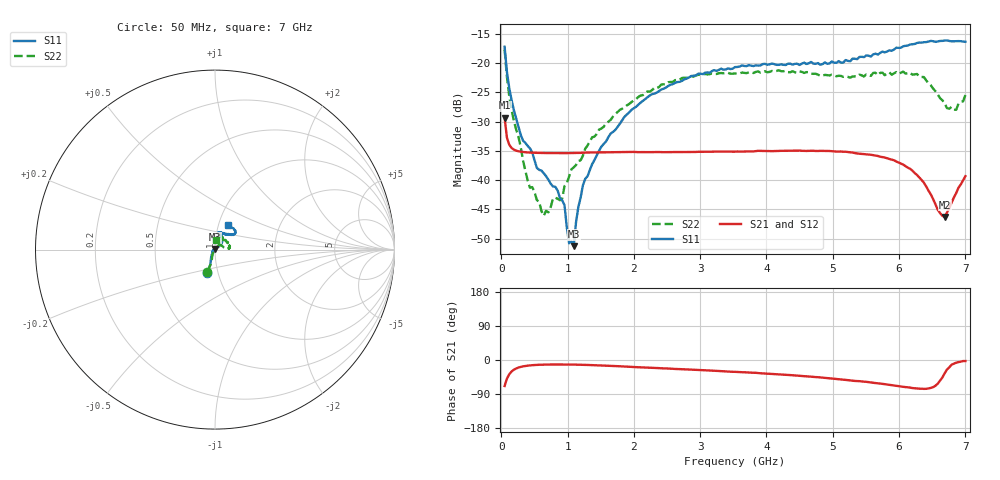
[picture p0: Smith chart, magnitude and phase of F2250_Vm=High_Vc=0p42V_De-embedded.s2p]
! Integrated Device Technology
! Corporate Headquarters
! 6024 Silver Creek Valley Road
! San Jose, CA 95138  USA
! Phone:  1-408-284-8200
! Toll Free:  1-800-223-1366
! Webpage:  http://www.idt.com/
! Timing and RF Division
! 515 Groton Road, Suite 102
! Westford, MA 01886-6024
! Device:  F2250
! Description: Voltage Variable RF Attenuator
! Frequency:  50.0 -  6000.00 MHz
! Package:  3x3 mm Thin QFN Plastic Package: 16 pin
! Ports:  2 RF, 3 DC
!  Pin  1  = GND
!  Pin  2  = NC
!  Pin  3  = RF1  = Port 1
!  Pin  4  = NC
!  Pin  5  = GND
!  Pin  6  = GND
!  Pin  7  = GND
!  Pin  8  = GND
!  Pin  9  = NC
!  Pin 10  = RF2  = Port 2
!  Pin 11  = NC
!  Pin 12  = GND
!  Pin 13  = GND
!  Pin 14  = VCNTRL
!  Pin 15  = VDD
!  Pin 16  = VMODE
! Vcntrl:  0.420 Volts
! Vmode:  +3.300 Volts
! Vdd:  +3.30  Volts
! Current:  1.265 mA
! Data:  The device was measured on a the F2250 evaluation board which has
!  individual transmission lines to the RF pins.  Data was collected
!  using a calibrated network analyzer.  The evaluation board was
!  de-embedded using a TRL calibration technique.
!  The reference plane is the edge of the package pin.
! Misc:  SN 10
!  Action Tracker AT0258
! Date Measured:  2014-11-26
! Date:  2015-10-15  MJV
! Note:
!  Integrated Device Technology supplies this data as a sample of measured
!  data at the package pin for this product.  Your particular data for this
!  product may vary.
!  Data was taken at 25 degrees C.
!  Integrated Device Technology reserves the right to change this data at anytime.
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# GHz S dB R 50
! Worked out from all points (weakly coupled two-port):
!   201 points, 50 MHz to 7 GHz, reference 50 ohm
!   highest |S21| = -29.30 dB at 50 MHz (marker M1); lowest = -46.3 dB at 6.687 GHz (marker M2)
!   lowest |S11| = -51.3 dB at 1.093 GHz (marker M3), VSWR 1.01, Z = 50 + j0.273 ohm
!   |S11| at or under -10 dB: start of sweep to end of sweep
!   |S22| runs from -46.1 to -17.7 dB; largest |S21 - S12| = 6.5e-05
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0.05  -17.17 -108.5  -29.30 -68.6  -29.30 -68.6  -17.67 -109.1
0.1195  -24.21 -112.0  -33.93 -37.7  -33.93 -37.6  -25.60 -108.8
0.29325  -32.26 -127.3  -35.13 -18.2  -35.13 -18.2  -34.35 -119.2
0.43225  -34.55 -145.3  -35.27 -14.2  -35.28 -14.2  -41.29 -155.1
0.5365  -37.90 -154.8  -35.32 -12.9  -35.32 -12.9  -43.40 -173.2
0.64075  -38.82 -162.5  -35.35 -12.2  -35.35 -12.2  -46.08 146.1
0.77975  -41.07 176.2  -35.37 -11.9  -35.37 -11.9  -43.12 115.9
0.91875  -43.45 156.1  -35.38 -11.9  -35.38 -11.9  -43.13 92.5
0.9535  -44.27 170.9  -35.37 -11.9  -35.38 -11.9  -41.00 95.3
1.023  -50.79 140.7  -35.36 -12.0  -35.37 -12.0  -39.36 77.6
1.0925  -51.28 89.6  -35.35 -12.2  -35.35 -12.2  -37.81 71.2
1.12725  -47.20 61.0  -35.34 -12.3  -35.34 -12.3  -37.40 64.3
1.2315  -40.86 40.2  -35.30 -12.7  -35.30 -12.7  -35.80 53.4
1.6485  -32.03 41.0  -35.22 -15.5  -35.22 -15.5  -29.69 48.4
2.37825  -24.75 46.6  -35.18 -21.4  -35.19 -21.4  -24.07 48.0
3.525  -20.65 71.7  -35.12 -31.2  -35.12 -31.2  -21.73 69.8
4.7065  -20.06 72.0  -34.97 -44.6  -34.97 -44.6  -21.81 68.5
5.85325  -17.79 40.5  -36.37 -65.4  -36.37 -65.5  -21.56 20.4
6.3745  -16.40 40.9  -40.44 -76.2  -40.45 -76.3  -22.36 4.1
6.68725  -16.11 47.9  -46.29 -35.0  -46.27 -34.6  -26.86 26.0
6.861  -16.22 54.5  -42.21 -7.1  -42.16 -7.1  -27.95 58.1
7  -16.33 62.4  -39.32 -2.7  -39.27 -2.9  -25.43 86.3
